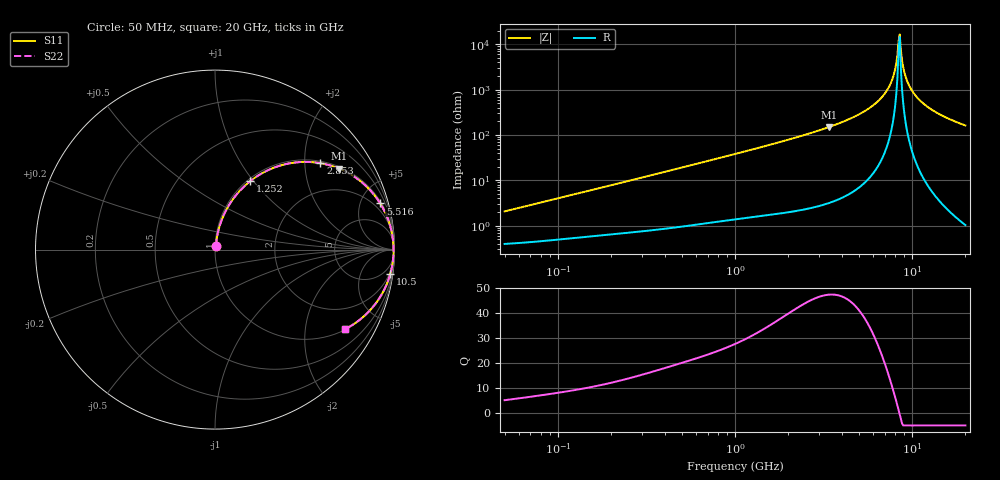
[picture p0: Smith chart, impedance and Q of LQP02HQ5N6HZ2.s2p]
!Murata Part Number: LQP02HQ5N6HZ2
!These Parameters are Measured in Series Mode Connection
!  o--[Z]--o
!Port1  Port2
!  o-------o
!Freq. Start=50[MHz] Stop=20[GHz], 401[Steps]
# Hz S RI R 50
!Freq.(Hz) S11(Real) S11(Imag) S21(Real) S21(Imag) S12(Real) S12(Imag) S22(Real) S22(Imag)
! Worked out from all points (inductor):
!   401 points, 50 MHz to 20 GHz, reference 50 ohm
!   read as one part in series: L = 6.44 nH near 51.52 MHz
!   highest Q = 47.4 at 3.415 GHz (marker M1), where L = 7.06 nH
!   self-resonance near 8.389 GHz
!   S11 on the Smith chart (normalised r, x): 50 MHz: 1.01, +0.04; 1.252 GHz: 1.03, +0.96; 2.853 GHz: 1.05, +2.39; 5.516 GHz: 1.19, +7.10; 10.5 GHz: 2, -15; 20 GHz: 1.02, -3.25
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5e7  0.00436 0.0202  0.9956 -0.0202  0.9956 -0.0202  0.00436 0.0202
1.364002e8  0.00839 0.0531  0.9916 -0.0531  0.9916 -0.0531  0.00839 0.0531
3.721004e8  0.0278 0.138  0.9722 -0.138  0.9722 -0.138  0.0278 0.138
1e9  0.1361 0.3253  0.8639 -0.3253  0.8639 -0.3253  0.1361 0.3253
1.251922e9  0.195 0.3804  0.805 -0.3804  0.805 -0.3804  0.195 0.3804
2.728004e9  0.5605 0.4854  0.4395 -0.4854  0.4395 -0.4854  0.5605 0.4854
2.853386e9  0.5871 0.4816  0.4129 -0.4816  0.4129 -0.4816  0.5871 0.4816
3.415248e9  0.6929 0.4509  0.3071 -0.4509  0.3071 -0.4509  0.6929 0.4509
5.515528e9  0.9205 0.2573  0.0795 -0.2573  0.0795 -0.2573  0.9205 0.2573
6.601595e9  0.9689 0.1546  0.0311 -0.1546  0.0311 -0.1546  0.9689 0.1546
7.442007e9  0.9875 0.0815  0.0125 -0.0815  0.0125 -0.0815  0.9875 0.0815
7.901521e9  0.9925 0.0442  0.00752 -0.0442  0.00752 -0.0442  0.9925 0.0442
8.264682e9  0.9944 0.016  0.00564 -0.016  0.00564 -0.016  0.9944 0.016
8.389408e9  0.9946 0.00656  0.00538 -0.00656  0.00538 -0.00656  0.9946 0.00656
8.516016e9  0.9947 -0.00286  0.00529 0.00286  0.00529 0.00286  0.9947 -0.00286
8.644534e9  0.9946 -0.0123  0.00538 0.0123  0.00538 0.0123  0.9946 -0.0123
9.041845e9  0.9933 -0.0405  0.00675 0.0405  0.00675 0.0405  0.9933 -0.0405
9.316812e9  0.9914 -0.0593  0.00855 0.0593  0.00855 0.0593  0.9914 -0.0593
9.745021e9  0.9874 -0.0873  0.0126 0.0873  0.0126 0.0873  0.9874 -0.0873
1.050288e10  0.9771 -0.1335  0.0229 0.1335  0.0229 0.1335  0.9771 -0.1335
1.354865e10  0.9095 -0.28  0.0905 0.28  0.0905 0.28  0.9095 -0.28
2e10  0.724 -0.4438  0.276 0.4438  0.276 0.4438  0.724 -0.4438
